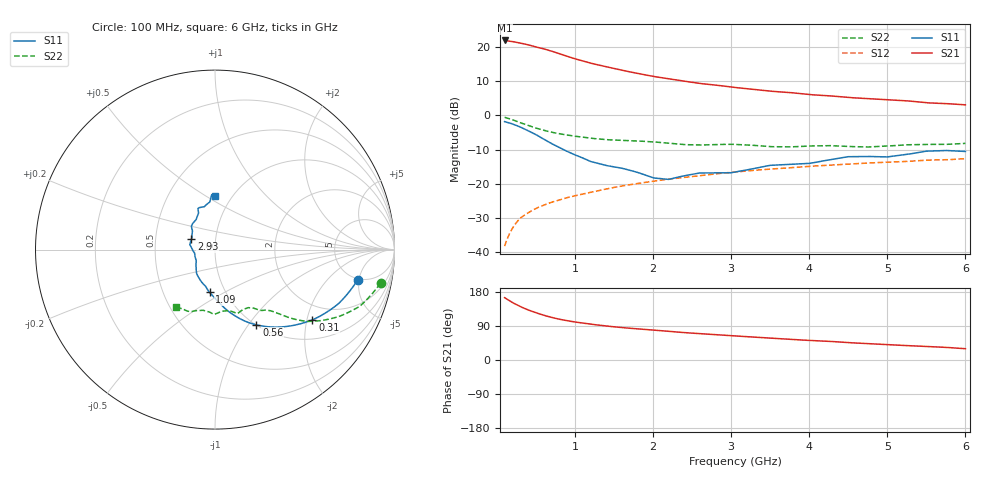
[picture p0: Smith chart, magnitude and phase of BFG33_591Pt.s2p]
! Created Thu Dec 04 15:46:49 2008  BFG33  591 Frequenzen
# mhz S ma R 50
! 2 Port Network Data from SP1.SP block
! freq  magS11  angS11  magS21  angS21  magS12  angS12  magS22  angS22
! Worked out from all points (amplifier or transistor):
!   591 points, 100 MHz to 6 GHz, reference 50 ohm
!   highest |S21| = 22.1 dB at 100 MHz (marker M1)
!   |S21| within 3 dB of that: start of sweep to 680.7 MHz
!   unconditionally stable (mu >= 1): 1.15 GHz to end of sweep
!   at 1.08 GHz: K = 0.97, MSG = 19.7 dB, |S12| = -23.2 dB
!   at 3.05 GHz: K = 1.25, MAG = 9.4 dB, |S12| = -16.6 dB
!   at 6 GHz: K = 1.36, MAG = 4.3 dB, |S12| = -12.7 dB
!   S11 on the Smith chart (normalised r, x): 100 MHz: 4.85, -4.80; 310 MHz: 1.53, -2.16; 560 MHz: 1.00, -1.09; 1.09 GHz: 0.84, -0.43; 2.93 GHz: 0.76, +0.09; 6 GHz: 0.84, +0.55
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100  0.813 -11.9  12.67 164.5  0.012 79.3  0.941 -11.5
120  0.8008 -14.2  12.58 161.9  0.014 77.8  0.9262 -13.5
140  0.7886 -16.5  12.49 159.3  0.016 76.4  0.9114 -15.4
210  0.7445 -24.6  12.16 150.5  0.0229 71.5  0.8587 -22.0
310  0.6689 -35.8  11.53 140.2  0.0316 66.9  0.777 -28.9
410  0.5888 -46.6  10.87 131.4  0.0376 63.6  0.708 -34.0
490  0.5312 -54.2  10.23 125.5  0.0424 62.0  0.66 -37.3
560  0.479 -61.1  9.795 120.8  0.046 61.4  0.6246 -39.3
670  0.4056 -70.6  9.05 114.1  0.0515 60.7  0.5791 -41.7
810  0.3339 -80.2  8.038 107.2  0.0575 60.4  0.5367 -43.6
940  0.2838 -87.7  7.17 102.3  0.0636 60.3  0.508 -44.9
1090  0.2402 -97.2  6.39 97.7  0.0696 60.3  0.4812 -46.4
1270  0.2016 -109.2  5.641 92.9  0.07715 60.1  0.4553 -48.3
1510  0.1752 -123.3  4.884 87.4  0.08795 59.9  0.435 -51.0
1790  0.1471 -135.5  4.174 82.6  0.0996 59.9  0.4224 -53.3
2070  0.1189 -156.3  3.65 77.8  0.1108 59.2  0.4033 -55.2
2580  0.1417 169.6  2.979 70.0  0.1302 57.2  0.3685 -64.4
2930  0.1436 156.5  2.681 65.0  0.1436 55.7  0.3766 -69.9
3050  0.1476 150.5  2.581 63.4  0.1478 55.4  0.3758 -71.0
4040  0.201 120.9  2.016 51.2  0.1801 51.5  0.3568 -88.9
5020  0.2477 103.6  1.696 40.6  0.2064 47.1  0.3563 -107.4
6000  0.296 89.6  1.434 29.8  0.232 42.9  0.389 -124.4
